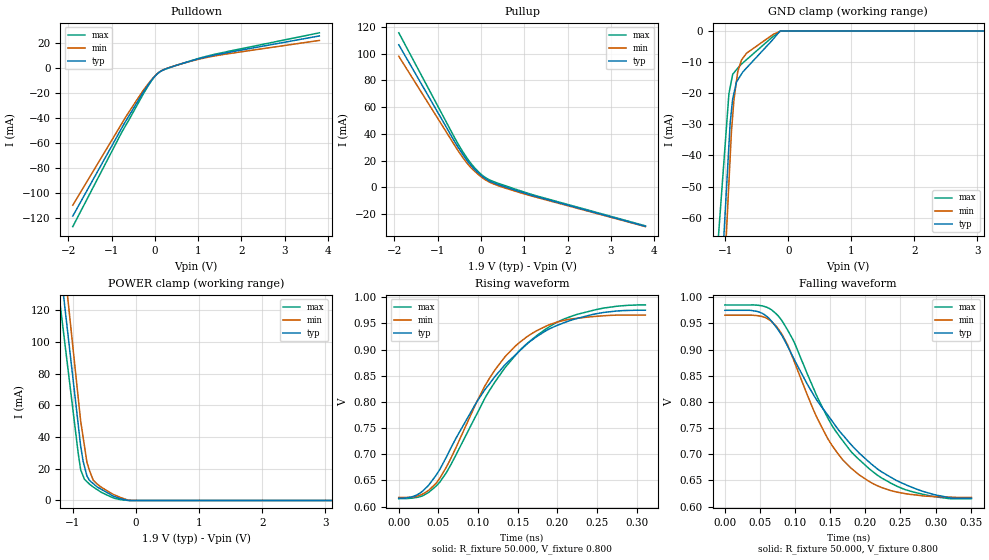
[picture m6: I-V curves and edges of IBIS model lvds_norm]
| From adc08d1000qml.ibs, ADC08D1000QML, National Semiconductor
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[Model]   lvds_norm
Model_type Output
Vref=8.000E-01
Rref=5.000E+01
Cref=2.500E-12
Vmeas=8.000E-01
C_comp   5.910E-13   5.910E-13   5.910E-13
[Voltage Range]   1.900E+00   1.800E+00   2.000E+00
[POWER Clamp Reference]   1.900E+00   1.800E+00   2.000E+00
[GND Clamp Reference]   0.000E+00   0.000E+00   0.000E+00
[Pullup Reference]   1.900E+00   1.800E+00   2.000E+00
[Pulldown Reference]   0.000E+00   0.000E+00   0.000E+00
[Temperature Range]   25   125   -55
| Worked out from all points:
|   slope of the pulldown table from 0 to 0.285 V, typ, clamps not added: 45.5 ohm
|   slope of the pullup table from 0 to 0.285 V, typ, clamps not added: 51 ohm
|   GND clamp passes 1 mA (typ) near -0.17 V on its own axis
|   POWER clamp passes 1 mA (typ) near -0.24 V on its own axis
|   rising waveform, R_fixture 50.000, V_fixture 0.800: 20-80 % time 98.8ps typ, 76.2ps min, 92.7ps max; typ from 0.616 V to 0.975 V
|   falling waveform, R_fixture 50.000, V_fixture 0.800: 20-80 % time 113ps typ, 76.4ps min, 92.1ps max; typ from 0.975 V to 0.616 V
[GND Clamp]
-2V       -423.4mA   -483.1mA   -312.6mA
-1.8V     -350.5mA   -401.2mA   -257.4mA
-940mV    -36.84mA   -48.8mA    -20.2mA
-920mV    -29.54mA   -40.6mA    -18.1mA
-900mV    -25.67mA   -32.41mA   -16mA
-860mV    -19.99mA   -22.06mA   -13.41mA
-800mV    -15.75mA   -13.08mA   -11.95mA
-740mV    -13.81mA   -9.307mA   -10.63mA
-660mV    -11.86mA   -7.124mA   -9.203mA
-240mV    -2.641mA   -1.106mA   -1.734mA
-130mV    0A         -92.15uA   -144.5uA
4V        0A         0A         0A
[Power Clamp]
-2.1V     461mA      513.7mA    417.7mA
-1.7V     321.1mA    361.8mA    286.4mA
-1V       76.46mA    95.81mA    56.5mA
-920mV    48.5mA     65.41mA    30.23mA
-880mV    34.52mA    50.21mA    19.48mA
-840mV    24.63mA    39.76mA    15.45mA
-780mV    15.46mA    24.07mA    11.88mA
-680mV    10.65mA    12.77mA    8.494mA
-560mV    7.227mA    8.585mA    5.346mA
-360mV    2.71mA     3.779mA    1.568mA
-120mV    0A         130uA      0A
3.9V      0A         0A         0A
[Pullup]
-1.9V     106.6mA    97.97mA    115.5mA
-620mV    34.77mA    31.97mA    37.7mA
-500mV    28.61mA    25.93mA    30.79mA
-240mV    16.68mA    14.98mA    18.17mA
-100mV    11.88mA    10.66mA    12.93mA
20mV      8.472mA    7.469mA    9.276mA
140mV     5.72mA     4.855mA    6.534mA
280mV     3.489mA    2.636mA    4.402mA
1.1V      -5.273mA   -5.884mA   -4.593mA
3.8V      -29.2mA    -29.37mA   -28.82mA
[Pulldown]
-1.9V     -118.6mA   -109.8mA   -127mA
-700mV    -43.73mA   -40.47mA   -47.22mA
-280mV    -19.72mA   -18.21mA   -21.23mA
-140mV    -12.47mA   -11.74mA   -13.16mA
-40mV     -7.842mA   -7.575mA   -8.079mA
80mV      -3.649mA   -3.635mA   -3.682mA
220mV     -888.1uA   -824.4uA   -985.5uA
440mV     1.772mA    1.815mA    1.712mA
1.3V      10.01mA    9.394mA    10.58mA
3.8V      25.95mA    22.35mA    28.45mA
[Rising Waveform]
R_fixture = 50.000
V_fixture = 0.800
V_fixture_min = 0.800
V_fixture_max = 0.800
|  time   V(typ)   V(min)   V(max)
0s        616mV      617.6mV    615.2mV
27.5ps    626.7mV    622.3mV    619.4mV
51ps      669.4mV    652.8mV    645.7mV
96ps      794.2mV    792.6mV    770mV
114ps     833.9mV    844.4mV    821.1mV
135ps     872.6mV    888.1mV    867.4mV
161.5ps   910.5mV    924.3mV    911.3mV
188ps     938mV      946.4mV    941.8mV
219.5ps   957.2mV    958.9mV    964.6mV
311ps     975.2mV    965.9mV    985.3mV
[Falling Waveform]
R_fixture = 50.000
V_fixture = 0.800
V_fixture_min = 0.800
V_fixture_max = 0.800
|  time   V(typ)   V(min)   V(max)
0s        975.2mV    965.9mV    985.3mV
48.5ps    972mV      964.4mV    984.6mV
76.5ps    936.7mV    938.9mV    963.7mV
97ps      886.1mV    883.4mV    918.9mV
126.5ps   813.1mV    783.7mV    825.3mV
146.5ps   775.1mV    730.1mV    769.6mV
190.5ps   703.4mV    661.4mV    690.6mV
256.5ps   642.6mV    625mV      632.7mV
301ps     622mV      619mV      618.6mV
351ps     616mV      617.6mV    615.2mV
[Ramp]
dV/dt_f   1.7616E+00/1.1244E-10   1.7022E+00/7.6000E-11   1.8220E+00/9.1820E-11
dV/dt_r   1.7616E+00/9.8650E-11   1.7022E+00/7.5950E-11   1.8220E+00/9.2600E-11
R_load = 50
